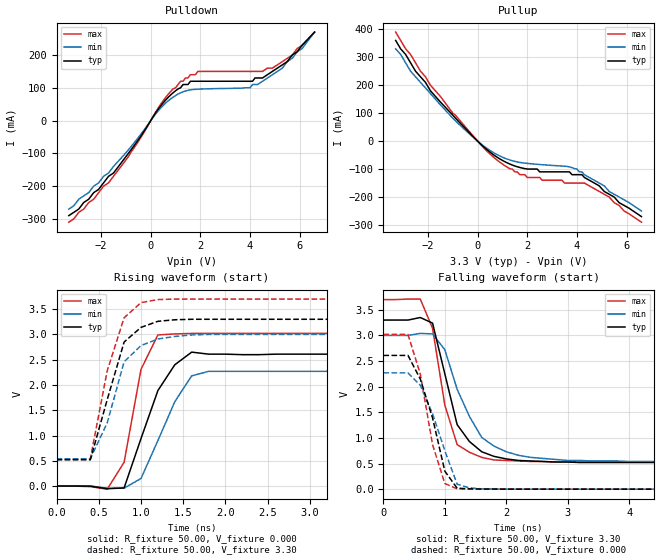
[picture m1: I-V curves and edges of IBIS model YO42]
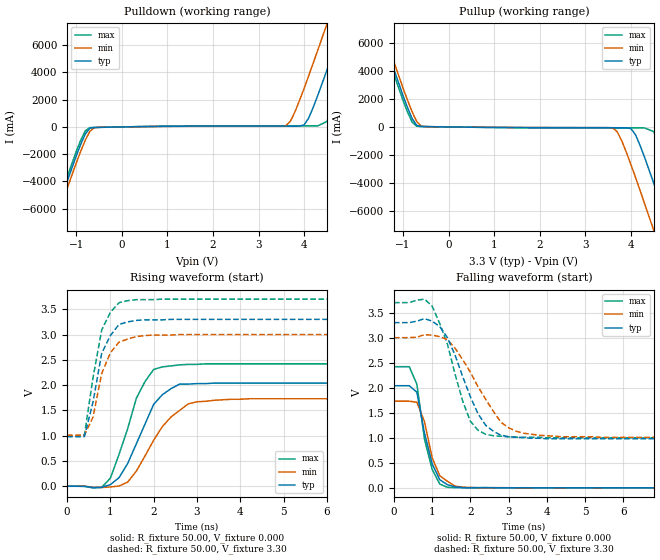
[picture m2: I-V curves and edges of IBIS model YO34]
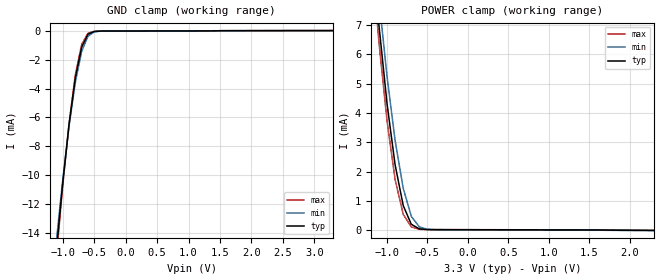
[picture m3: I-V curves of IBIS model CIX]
|   * 952601e.ibs * IBIS 2.1 Model file
| Components:
| ICS952601e   CK409 CLOCK
| Rev History
| Rev No.   Description
| 1.0   Initial release with Updated Parasitic Parameters
| 1.1   ibis revisit
| 1.2   Update USB model
| 1.3   Update USB model added 2xUSB48 model
[IBIS Ver]   2.1
[Comment char]  |_char
[File name]   952601e.ibs
[Date]   April 8, 2003
[File Rev]   1.3
[Source]   Originated at Integrated Circuit Systems, Inc.
[Disclaimer] (C) Copyright Integrated Circuit Systems, Inc. 2002
   All rights reserved
ICS hereby grants the user of this IBIS model a non-exclusive,
nontransferable license to use this IBIS model under the following terms.
Before using this IBIS model, the user should read this license.
If the user does not accept these terms,  the IBIS model should be
returned to ICS within 30 days.
   The user is granted this license only to use the IBIS model and
is not granted rights to sell, load, rent, lease or license the IBIS
model in whole or in part, or in modified form to anyone other than
user. User may modify the IBIS model to suit its specific
applications but rights to derivative works and such modifications
shall belong to ICS.
   This IBIS model is provided on an "AS IS" basis and ICS makes
absolutely no warranty with respect to the information contained
herein. ICS DISCLAIMS AND CUSTOMER WAIVES ALL WARRANTIES, EXPRESS
OR IMPLIED, INCLUDING WARRANTIES OF MERCHANTABILITY OR FITNESS FOR
A PARTICULAR PURPOSE. The entire risk as to quality and performance
is with the Customer. ACCORDINGLY, IN NO EVENT SHALL THE COMPANY BE
LIABLE FOR ANY DAMAGES, WHETHER IN CONTRACT OR TORT,INCLUDING ANY
LOST PROFITS OR OTHER INCIDENTAL, CONSEQUENTIAL, EXEMPLARY, OR
PUNITIVE DAMAGES ARISING OUT OF THE USE OR APPLICATION OF THE IBIS
model provided in this package. Further, ICS reserves the right to
make changes without notice to any product herein to improve
reliability, function, or design. ICS does not convey any license
under patent rights or any other intellectual property rights,
including those of third parties.
   ICS is not obligated to provide maintenance or support
for the licensed IBIS model.
|   COMPONENT: ICS952601e
[Component]   ICS952601e
[Manufacturer]  ICS
[Package]
| variable   typ   min   max
R_pkg   81.1m   62.2m   100.0m
L_pkg   6.7nH   4.9nH   8.5nH
C_pkg   0.53pF  0.21pF  0.85pF
[Pin]   signal_name   model_name   R_pin   L_pin   C_pin
  1   REF0   YO34
  2   REF1   YO34
  3   VDDREF   POWER
  4   X1   CIX
  5   X2   CIX
  6   GND   GND
  7   PCICLK_F0   YO34
  8   PCICLK_F1   YO34
  9   PCICLK_F2   YO34
 10   VDDPCI   POWER
 11   GND   GND
 12   PCICLK0   YO34
 13   PCICLK1   YO34
 14   PCICLK2   YO34
 15   PCICLK3   YO34
 16   VDDPCI   POWER
 17   GND   GND
 18   PCICLK4   YO34
 19   PCICLK5   YO34
 20   PCICLK6   YO34
 21   PD#   YI3
 22   3V66_0   YO35
 23   3V66_1   YO35
 24   VDD3V66   POWER
 25   GND   GND
 26   3V66_2   YO35
 27   3V66_3   YO35
 28   SCLK   CI3
 29   3V66_4/VCH   YO36
 30   SDATA   XIOD1
 31   48MHz_USB   YO34
 32   48MHz_DOT   YO33
 33   GND   GND
 34   VDD48   POWER
 35   Vtt_PWRGD#   CI10
 36   VDD   POWER
 37   SRCCLKC   YO32
 38   SRCCLKT   YO32
 39   GND   GND
 40   CPUCLKC0   YO32
 41   CPUCLKT0   YO32
 42   VDDCPU   POWER
 43   CPUCLKC1   YO32
 44   CPUCLKT1   YO32
 45   GND   GND
 46   CPUCLKC2   YO32
 47   CPUCLKT2   YO32
 48   VDDCPU   POWER
 49   PCI_STOP#   YI1
 50   CPU_STOP#   YI2
 51   FS_A   CI4
 52   IREF   CI10
 53   GND   GND
 54   GNDA   GND
 55   VDDA   POWER
 56   FS_B   CI11
|* Either 3.3V or 2.5V
|** All model are simulated with typical corner process
[Diff Pin]   inv_pin   vdiff   tdelay_typ
38   37   NA   NA
41   40   NA   NA
44   43   NA   NA
47   46   NA   NA
|   COMPONENT: ICS952601e_usb48x2
[Component]   ICS952601e_usb48x2
[Manufacturer]  ICS
[Package]
| variable   typ   min   max
R_pkg   81.1m   62.2m   100.0m
L_pkg   6.7nH   4.9nH   8.5nH
C_pkg   0.53pF  0.21pF  0.85pF
[Pin]   signal_name   model_name   R_pin   L_pin   C_pin
  1   REF0   YO34
  2   REF1   YO34
  3   VDDREF   POWER
  4   X1   CIX
  5   X2   CIX
  6   GND   GND
  7   PCICLK_F0   YO34
  8   PCICLK_F1   YO34
  9   PCICLK_F2   YO34
 10   VDDPCI   POWER
 11   GND   GND
 12   PCICLK0   YO34
 13   PCICLK1   YO34
 14   PCICLK2   YO34
 15   PCICLK3   YO34
 16   VDDPCI   POWER
 17   GND   GND
 18   PCICLK4   YO34
 19   PCICLK5   YO34
 20   PCICLK6   YO34
 21   PD#   YI3
 22   3V66_0   YO35
 23   3V66_1   YO35
 24   VDD3V66   POWER
 25   GND   GND
 26   3V66_2   YO35
 27   3V66_3   YO35
 28   SCLK   CI3
 29   3V66_4/VCH   YO36
 30   SDATA   XIOD1
 31   48MHz_USB   YO42
 32   48MHz_DOT   YO33
 33   GND   GND
 34   VDD48   POWER
 35   Vtt_PWRGD#   CI10
 36   VDD   POWER
 37   SRCCLKC   YO32
 38   SRCCLKT   YO32
 39   GND   GND
 40   CPUCLKC0   YO32
 41   CPUCLKT0   YO32
 42   VDDCPU   POWER
 43   CPUCLKC1   YO32
 44   CPUCLKT1   YO32
 45   GND   GND
 46   CPUCLKC2   YO32
 47   CPUCLKT2   YO32
 48   VDDCPU   POWER
 49   PCI_STOP#   YI1
 50   CPU_STOP#   YI2
 51   FS_A   CI4
 52   IREF   CI10
 53   GND   GND
 54   GNDA   GND
 55   VDDA   POWER
 56   FS_B   CI11
|* Either 3.3V or 2.5V
|** All model are simulated with typical corner process
[Diff Pin]   inv_pin   vdiff   tdelay_typ
38   37   NA   NA
41   40   NA   NA
44   43   NA   NA
47   46   NA   NA
| Models and submodels in the file (15): YO42 (Output), YO34 (Output), CIX (Input), YI3 (Input), CI3 (Input), YO35 (Output), YO36 (Output), XIOD1 (I/O_open_drain), YO33 (Output), CI10 (Input), YO32 (Open_source), YI1 (Input), YI2 (Input), CI4 (Input), CI11 (Input)
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|   Model YO42
[Model]   YO42
Model_type   Output
Polarity   Non-Inverting
Vmeas =   1.50V
Cref =  20.00pF
Rref =  0.000
Vref =   1.50V
C_comp   5.50pF   5.00pF   6.00pF
[Temperature Range]   27.00   70.00   0.000
[Voltage Range]   3.30V   3.00V   3.70V
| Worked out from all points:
|   slope of the pulldown table from 0 to 0.495 V, typ, clamps not added: 9.26 ohm
|   slope of the pullup table from 0 to 0.495 V, typ, clamps not added: 12.6 ohm
|   rising waveform, R_fixture 50.00, V_fixture 0.000: 20-80 % time 363ps typ, 376ps min, 217ps max; typ from 0 V to 2.61 V
|   rising waveform, R_fixture 50.00, V_fixture 3.30: 20-80 % time 288ps typ, 291ps min, 278ps max; typ from 0.52 V to 3.3 V
|   falling waveform, R_fixture 50.00, V_fixture 3.30: 20-80 % time 411ps typ, 534ps min, 314ps max; typ from 3.3 V to 0.52 V
|   falling waveform, R_fixture 50.00, V_fixture 0.000: 20-80 % time 351ps typ, 414ps min, 313ps max; typ from 2.61 V to 0 V
[Pulldown]
| voltage   I(typ)   I(min)   I(max)
-3.3V     -290mA     -270mA     -310mA
-2.9V     -270mA     -240mA     -280mA
-1.7V     -170mA     -160mA     -190mA
-800mV    -89.75mA   -80.1mA    -97.28mA
400mV     44.59mA    38.34mA    49.72mA
1.2V      100mA      84.58mA    120mA
1.9V      120mA      95.81mA    150mA
4.1V      120mA      110mA      150mA
4.3V      130mA      110mA      150mA
4.9V      150mA      140mA      160mA
5.5V      180mA      180mA      190mA
6.6V      270mA      270mA      270mA
[Pullup]
| voltage   I(typ)   I(min)   I(max)
-3.3V     360mA      330mA      390mA
-2.7V     280mA      250mA      310mA
-1.9V     180mA      170mA      200mA
-400mV    36.41mA    31.65mA    41.28mA
800mV     -58.4mA    -49.04mA   -68.76mA
2V        -99.81mA   -79.7mA    -130mA
3.4V      -110mA     -89.19mA   -140mA
3.6V      -110mA     -90.59mA   -150mA
4.2V      -120mA     -110mA     -150mA
5.3V      -190mA     -180mA     -200mA
5.9V      -230mA     -210mA     -250mA
6.6V      -270mA     -250mA     -290mA
[Ramp]
| variable   typ   min   max
dV/dt_r   1.56/0.32n   1.36/0.29n   1.81/0.18n
dV/dt_f   1.67/0.35n   1.48/0.47n   1.90/0.27n
R_load = 50.00
[Rising Waveform]
R_fixture = 50.00
V_fixture = 0.000
V_fixture_min = 0.000
V_fixture_max = 0.000
| time   V(typ)   V(min)   V(max)
0s        0V         100uV      200uV
400ps     -2.15mV    990uV      -11.71mV
600ps     -53.2mV    -42.12mV   -61.72mV
800ps     -37.13mV   -41.7mV    470mV
1ns       940mV      150mV      2.31V
1.2ns     1.89V      900mV      2.99V
1.4ns     2.4V       1.67V      3.01V
1.6ns     2.65V      2.18V      3.02V
1.8ns     2.61V      2.27V      3.02V
10ns      2.61V      2.27V      3.02V
[Rising Waveform]
R_fixture = 50.00
V_fixture = 3.30
V_fixture_min = 3.00
V_fixture_max = 3.70
| time   V(typ)   V(min)   V(max)
0s        520mV      540mV      530mV
400ps     520mV      540mV      540mV
600ps     1.71V      1.25V      2.28V
800ps     2.85V      2.46V      3.33V
1ns       3.14V      2.78V      3.63V
1.2ns     3.26V      2.91V      3.69V
1.4ns     3.29V      2.96V      3.7V
1.6ns     3.3V       2.99V      3.7V
1.8ns     3.3V       3V         3.7V
10ns      3.3V       3V         3.7V
[Falling Waveform]
R_fixture = 50.00
V_fixture = 3.30
V_fixture_min = 3.00
V_fixture_max = 3.70
| time   V(typ)   V(min)   V(max)
0s        3.3V       3V         3.7V
600ps     3.35V      3.04V      3.71V
800ps     3.24V      3.03V      3.14V
1ns       2.25V      2.72V      1.64V
1.2ns     1.26V      1.95V      870mV
1.4ns     930mV      1.42V      720mV
1.6ns     730mV      1.01V      620mV
2.2ns     560mV      660mV      550mV
3ns       530mV      560mV      530mV
10ns      520mV      540mV      530mV
[Falling Waveform]
R_fixture = 50.00
V_fixture = 0.000
V_fixture_min = 0.000
V_fixture_max = 0.000
| time   V(typ)   V(min)   V(max)
0s        2.61V      2.27V      3.02V
400ps     2.61V      2.27V      3.02V
600ps     2.15V      2.03V      2.25V
800ps     1.39V      1.47V      870mV
1ns       350mV      750mV      110mV
1.2ns     19.13mV    96.46mV    7.14mV
1.4ns     6.49mV     26.04mV    3.27mV
1.8ns     1.97mV     2.78mV     1.59mV
10ns      8.22uV     -1.22uV    0V
|   Model YO34
[Model]   YO34
Model_type   Output
Polarity   Non-Inverting
C_comp   5.50pF   5.00pF   6.00pF
[Temperature Range]   27.00   70.00   0.000
[Voltage Range]   3.30V   3.00V   3.70V
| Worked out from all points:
|   slope of the pulldown table from 0 to 0.495 V, typ, clamps not added: 18 ohm
|   slope of the pullup table from 0 to 0.495 V, typ, clamps not added: 25.6 ohm
|   rising waveform, R_fixture 50.00, V_fixture 0.000: 20-80 % time 643ps typ, 791ps min, 581ps max; typ from 0 V to 2.04 V
|   rising waveform, R_fixture 50.00, V_fixture 3.30: 20-80 % time 383ps typ, 373ps min, 347ps max; typ from 0.98 V to 3.3 V
|   falling waveform, R_fixture 50.00, V_fixture 0.000: 20-80 % time 377ps typ, 374ps min, 338ps max; typ from 2.04 V to 0 V
|   falling waveform, R_fixture 50.00, V_fixture 3.30: 20-80 % time 738ps typ, 947ps min, 636ps max; typ from 3.3 V to 0.98 V
[Pulldown]
| voltage   I(typ)   I(min)   I(max)
-3.3V     -24.5A     -25.12A    -24.2A
-1.7V     -8.77A     -9.29A     -8.45A
-1.5V     -6.83A     -7.35A     -6.51A
-900mV    -1.27A     -1.78A     -970mA
-700mV    -92.33mA   -320mA     -53mA
3.6V      62.06mA    88.77mA    76.48mA
4V        150mA      2.83A      76.72mA
4.3V      2.31A      5.64A      77.26mA
4.5V      4.16A      7.55A      400mA
4.9V      8A         11.44A     3.83A
5.3V      11.9A      15.36A     7.68A
6.6V      24.75A     28.22A     20.49A
[Pullup]
| voltage   I(typ)   I(min)   I(max)
-3.3V     24.61A     25.12A     24.3A
-1.7V     8.88A      9.42A      8.55A
-1.5V     6.94A      7.49A      6.61A
-900mV    1.37A      1.9A       1.05A
-700mV    110mA      380mA      48.51mA
3.6V      -57.33mA   -72.21mA   -72.12mA
3.8V      -57.8mA    -1.01A     -72.62mA
4.1V      -560mA     -3.62A     -73.3mA
4.5V      -4.04A     -7.42A     -340mA
4.9V      -7.88A     -11.31A    -3.72A
5.3V      -11.78A    -15.23A    -7.57A
6.6V      -24.64A    -28.1A     -20.38A
[Ramp]
| variable   typ   min   max
dV/dt_r   1.23/0.63n   1.04/0.78n   1.45/0.50n
dV/dt_f   1.39/0.73n   1.19/0.94n   1.62/0.58n
R_load = 50.00
[Rising Waveform]
R_fixture = 50.00
V_fixture = 0.000
V_fixture_min = 0.000
V_fixture_max = 0.000
| time   V(typ)   V(min)   V(max)
0s        0V         130uV      260uV
800ps     -21.29mV   -24.18mV   -20.91mV
1ns       32.3mV     -13.99mV   160mV
1.2ns     170mV      5.7mV      630mV
1.6ns     840mV      300mV      1.74V
2ns       1.62V      910mV      2.31V
2.2ns     1.81V      1.18V      2.36V
2.8ns     2.02V      1.63V      2.41V
3.4ns     2.04V      1.7V       2.42V
10ns      2.04V      1.73V      2.42V
[Rising Waveform]
R_fixture = 50.00
V_fixture = 3.30
V_fixture_min = 3.00
V_fixture_max = 3.70
| time   V(typ)   V(min)   V(max)
0s        980mV      1.01V      1V
400ps     980mV      1.01V      1.01V
600ps     1.67V      1.37V      2.15V
800ps     2.63V      2.23V      3.09V
1ns       2.98V      2.64V      3.44V
1.2ns     3.2V       2.85V      3.63V
1.4ns     3.25V      2.91V      3.67V
1.6ns     3.28V      2.96V      3.69V
2ns       3.29V      2.99V      3.69V
10ns      3.3V       3V         3.7V
[Falling Waveform]
R_fixture = 50.00
V_fixture = 0.000
V_fixture_min = 0.000
V_fixture_max = 0.000
| time   V(typ)   V(min)   V(max)
0s        2.04V      1.73V      2.42V
400ps     2.04V      1.73V      2.42V
600ps     1.91V      1.71V      2.07V
800ps     1.09V      1.32V      970mV
1ns       480mV      600mV      370mV
1.2ns     160mV      240mV      74.26mV
1.4ns     60.86mV    130mV      10.1mV
1.6ns     17.76mV    33.58mV    2.93mV
2.2ns     2.17mV     1.49mV     1.69mV
10ns      2.03uV     -5.17uV    -710nV
[Falling Waveform]
R_fixture = 50.00
V_fixture = 3.30
V_fixture_min = 3.00
V_fixture_max = 3.70
| time   V(typ)   V(min)   V(max)
0s        3.3V       3V         3.7V
800ps     3.38V      3.06V      3.77V
1ns       3.33V      3.05V      3.63V
1.4ns     3V         2.96V      2.87V
1.8ns     2.22V      2.56V      1.73V
2ns       1.82V      2.31V      1.33V
2.4ns     1.25V      1.77V      1.07V
2.8ns     1.05V      1.31V      1.03V
3.4ns     1V         1.09V      1.01V
10ns      980mV      1.01V      1V
|   Model CIX
[Model]   CIX
Model_type   Input
Polarity   Non-Inverting
Vinl =   0.80V
Vinh =   2.00V
C_comp   5.50pF   5.00pF   6.00pF
[Temperature Range]   27.00   70.00   0.000
[Voltage Range]   3.30V   3.00V   3.70V
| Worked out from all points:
|   GND clamp passes 1 mA (typ) near -0.69 V on its own axis
|   POWER clamp passes 1 mA (typ) near -0.81 V on its own axis
[GND_clamp]
| voltage   I(typ)   I(min)   I(max)
-3.3V     -140mA     -130mA     -150mA
-1.1V     -15.06mA   -14.43mA   -15.54mA
-1V       -10.47mA   -10.26mA   -10.64mA
-900mV    -6.45mA    -6.56mA    -6.37mA
-800mV    -3.23mA    -3.53mA    -3.01mA
-700mV    -1.13mA    -1.42mA    -940uA
-600mV    -240uA     -380uA     -170uA
-500mV    -45.93uA   -76.06uA   -35.4uA
-400mV    -20.06uA   -23.55uA   -20.53uA
3.3V      15.02uA    15.15uA    15.02uA
[POWER_clamp]
| voltage   I(typ)   I(min)   I(max)
-3.3V     150mA      140mA      150mA
-1.2V     10.13mA    10.93mA    9.65mA
-1.1V     6.98mA     7.88mA     6.4mA
-1V       4.31mA     5.24mA     3.72mA
-900mV    2.22mA     3.05mA     1.72mA
-800mV    840uA      1.43mA     540uA
-700mV    200uA      470uA      110uA
-600mV    42.64uA    110uA      28.63uA
-500mV    19.91uA    29.2uA     20uA
2.3V      -10.4uA    -10.91uA   -6.15uA
